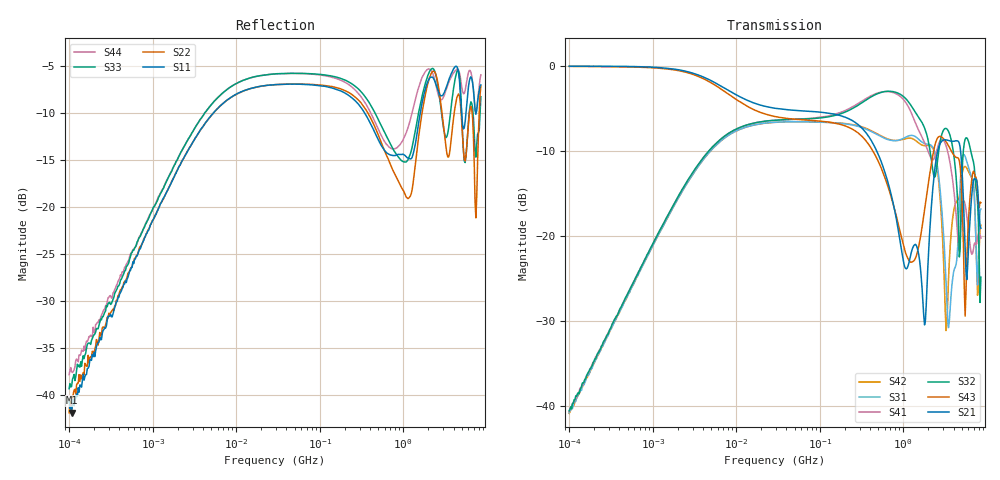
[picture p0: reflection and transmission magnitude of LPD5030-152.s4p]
# MHz S MA R 50
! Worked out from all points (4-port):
!   498 points, 100 kHz to 8.5 GHz, reference 50 ohm
!   strongest paths, dB at 100 kHz, 1.698 MHz, 29.49 MHz, 500.7 MHz, 8.5 GHz:
!     S21: -0.1, -0.4, -5.0, -10.4, -19.1
!     S43: -0.1, -0.4, -6.0, -11.2, -16.1
!     S32: -40.5, -16.7, -6.4, -3.3, -24.8
!     S41: -40.6, -16.7, -6.4, -3.2, -20.3
!     S31: -40.8, -16.9, -6.6, -8.2, -16.8
!     S42: -40.8, -16.9, -6.6, -8.1, -18.7
!   lowest |S11| = -41.9 dB at 107.1 kHz (marker M1), VSWR 1.02, Z = 50.1 + j0.799 ohm
!   |S11| at or under -10 dB: start of sweep to 5.377 MHz; 343 MHz to 1.601 GHz (1.258 GHz wide, 129 % of centre); 4.993 GHz to 5.641 GHz (648.6 MHz wide, 12.2 % of centre)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
0.1  0.009185 85.1  0.994 -0.5  0.009148 -89.1  0.009292 90.3
     0.994 -0.5  0.008003 86.0  0.009395 88.9  0.009076 -93.4
     0.009148 -89.1  0.009395 88.9  0.01076 75.7  0.9916 -0.7
     0.009292 90.3  0.009076 -93.4  0.9916 -0.7  0.01278 85.1
0.1070915  0.00804 82.9  0.9938 -0.5  0.009667 -92.4  0.01002 88.8
           0.9938 -0.5  0.007964 87.9  0.009632 89.4  0.009758 -91.6
           0.009667 -92.4  0.009632 89.4  0.01107 75.9  0.9918 -0.8
           0.01002 88.8  0.009758 -91.6  0.9918 -0.8  0.01324 80.4
13.25948  0.418 19.5  0.6299 -18.2  0.4368 -161.9  0.4482 21.2
          0.6299 -18.2  0.4173 19.4  0.4484 21.3  0.4366 -161.9
          0.4368 -161.9  0.4484 21.3  0.4767 19.5  0.5821 -21.7
          0.4482 21.2  0.4366 -161.9  0.5821 -21.7  0.4763 19.3
643.6438  0.1922 -95.1  0.2132 -153.1  0.3694 2.5  0.7051 -96.7
          0.2132 -153.1  0.1838 -115.9  0.7081 -91.2  0.3722 -0.9
          0.3694 2.5  0.7081 -91.2  0.2325 -108.4  0.2009 -163.7
          0.7051 -96.7  0.3722 -0.9  0.2009 -163.7  0.2126 -95.3
1798.752  0.4079 156.2  0.03002 3.5  0.3495 135.2  0.3537 81.3
          0.03002 3.5  0.3744 156.7  0.4312 83.9  0.3391 135.9
          0.3495 135.2  0.4312 83.9  0.437 139.1  0.1419 -76.0
          0.3537 81.3  0.3391 135.9  0.1419 -76.0  0.5144 140.1
4383.155  0.5555 -178.2  0.3622 152.7  0.07296 -146.0  0.117 79.0
          0.3622 152.7  0.3802 -154.6  0.1927 91.1  0.1599 -179.2
          0.07296 -146.0  0.1927 91.1  0.5215 -170.9  0.2885 153.9
          0.117 79.0  0.1599 -179.2  0.2885 153.9  0.5386 -178.9
8500  0.4438 -37.6  0.1108 -17.3  0.1441 -2.8  0.09713 103.9
      0.1108 -17.3  0.4376 -31.8  0.05724 -81.8  0.1158 -0.7
      0.1441 -2.8  0.05724 -81.8  0.3838 -23.8  0.1569 -17.6
      0.09713 103.9  0.1158 -0.7  0.1569 -17.6  0.5021 -41.2
